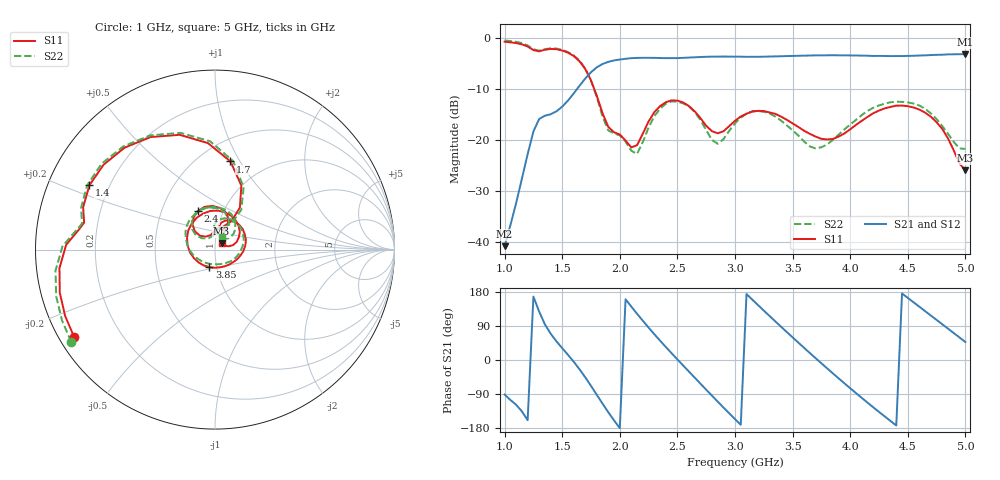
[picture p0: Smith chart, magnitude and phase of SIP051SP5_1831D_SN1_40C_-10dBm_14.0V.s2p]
# GHz  S  dB  R  50
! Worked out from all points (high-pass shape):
!   81 points, 1 GHz to 5 GHz, reference 50 ohm
!   highest |S21| = -3.11 dB at 5 GHz (marker M1); lowest = -40.9 dB at 1 GHz (marker M2)
!   |S21| within 3 dB of the highest: 1.779 GHz to end of sweep
!   lowest |S11| = -26.0 dB at 5 GHz (marker M3), VSWR 1.11, Z = 53.7 + j3.71 ohm
!   |S11| at or under -10 dB: 1.779 GHz to end of sweep
!   |S22| runs from -22.8 to -0.4 dB; largest |S21 - S12| = 0.0019
!   S11 on the Smith chart (normalised r, x): 1 GHz: 0.04, -0.29; 1.4 GHz: 0.13, +0.24; 1.7 GHz: 0.70, +0.91; 2.4 GHz: 0.76, +0.35; 3.85 GHz: 0.92, -0.18; 5 GHz: 1.07, +0.07
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1  -0.69 -148.0  -40.91 -91.2  -40.90 -92.9  -0.42 -147.3
1.25  -2.32 171.6  -18.34 167.4  -18.34 167.7  -2.15 172.2
1.4  -2.09 152.9  -14.95 69.3  -14.94 69.4  -1.97 153.2
1.55  -2.82 119.8  -12.26 13.7  -12.25 13.7  -2.72 119.5
1.7  -6.04 80.0  -7.92 -45.7  -7.93 -45.7  -5.96 78.5
1.85  -14.75 59.8  -5.06 -115.0  -5.04 -115.1  -15.39 57.8
2  -18.93 89.0  -4.18 -179.9  -4.17 -179.9  -19.10 88.7
2.2  -18.77 137.4  -3.84 103.5  -3.83 103.4  -20.40 138.8
2.35  -13.32 123.4  -3.89 50.8  -3.88 50.9  -13.84 129.1
2.4  -12.57 113.9  -3.90 34.1  -3.91 34.1  -12.88 118.7
2.55  -12.62 83.3  -3.85 -14.5  -3.85 -14.5  -12.79 85.4
2.75  -17.22 61.6  -3.64 -78.4  -3.64 -78.4  -18.07 59.1
3  -16.24 76.9  -3.61 -156.0  -3.60 -156.0  -16.75 90.3
3.15  -14.42 55.4  -3.64 159.3  -3.64 159.4  -14.36 64.3
3.35  -14.87 17.1  -3.57 101.9  -3.57 101.9  -15.41 19.0
3.5  -16.75 -13.4  -3.47 59.8  -3.48 59.8  -18.11 -21.3
3.7  -19.35 -60.0  -3.37 4.7  -3.37 4.9  -21.66 -89.8
3.85  -19.81 -107.7  -3.33 -35.4  -3.34 -35.4  -20.01 -141.8
4.1  -16.24 171.8  -3.40 -99.9  -3.40 -99.9  -15.11 158.3
4.35  -13.50 108.1  -3.50 -160.9  -3.50 -161.0  -12.58 110.3
4.7  -15.42 35.3  -3.30 117.4  -3.30 117.4  -14.78 51.7
5  -25.95 43.1  -3.12 47.5  -3.12 47.6  -21.77 60.5
